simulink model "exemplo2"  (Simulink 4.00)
settings: Solver=ode45  StartTime=0.0  StopTime=10  MaxStep=0.1  RelTol=1e-4
libraries: simulink_extras x1

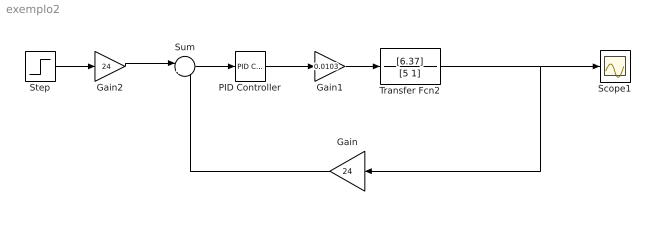
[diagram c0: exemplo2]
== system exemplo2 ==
  Gain : Gain  Orientation=left  Gain=24  Multiplication=Element-wise(K.*u)  SaturateOnIntegerOverflow=on
  Gain1 : Gain  Gain=0.0103  Multiplication=Element-wise(K.*u)  SaturateOnIntegerOverflow=on
  Gain2 : Gain  Gain=24  Multiplication=Element-wise(K.*u)  SaturateOnIntegerOverflow=on
  PID Controller : simulink_extras/Additional Linear/PID Controller  P=2  I=0  D=0
  Scope1 : Scope
  Step : Step  Time=0  Before=0  After=1  SampleTime=0
  Sum : Sum  Inputs=|+-  SaturateOnIntegerOverflow=on
  Transfer Fcn2 : TransferFcn  Numerator=[6.37]  Denominator=[5 1]  AbsoluteTolerance=auto  Realization=auto
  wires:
  Sum/1 -> PID Controller/1
  PID Controller/1 -> Gain1/1
  Gain1/1 -> Transfer Fcn2/1
  Gain/1 -> Sum/2
  Transfer Fcn2/1 -> Gain/1, Scope1/1
  Step/1 -> Gain2/1
  Gain2/1 -> Sum/1
